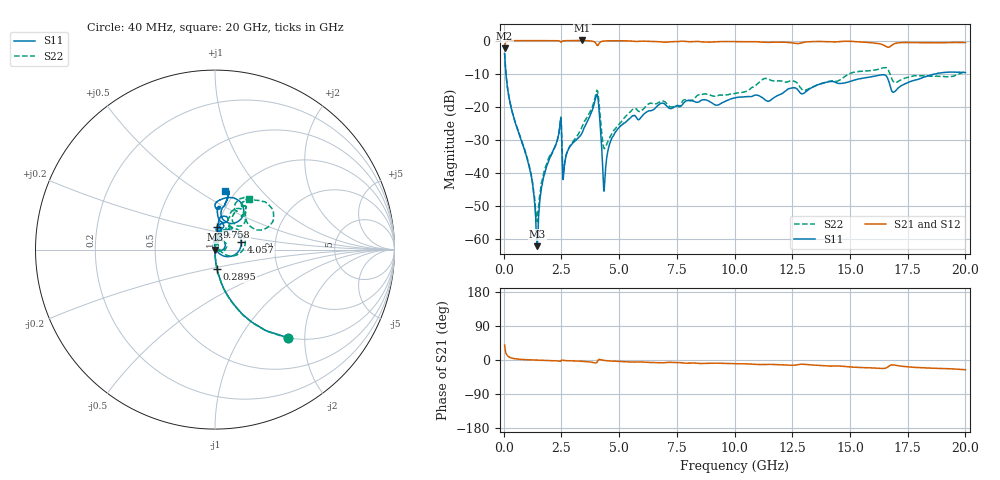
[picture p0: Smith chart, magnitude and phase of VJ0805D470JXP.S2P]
! VJ0805D470JXP
! DATE 10/29/2021  12:48
! CAPACITORS MOUNTED IN SERIES ON 25 MIL THICK MICROSTRIP SUBSTRATE
# GHz  S  MA  R  50.00
!  FREQ  S11M  S11A  S21M  S21A  S12M  S12A  S22M  S22A
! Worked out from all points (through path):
!   1601 points, 40 MHz to 20 GHz, reference 50 ohm
!   highest |S21| = 0.04 dB at 3.408 GHz (marker M1); lowest = -2.3 dB at 40 MHz (marker M2)
!   group delay of S21, straight-line fit = 3.63 ps
!   lowest |S11| = -62.0 dB at 1.462 GHz (marker M3), VSWR 1.00, Z = 49.9 + j0.0319 ohm
!   |S11| at or under -10 dB: 99.02 MHz to 18.74 GHz (18.64 GHz wide, 198 % of centre)
!   |S22| runs from -54.6 to -3.9 dB; largest |S21 - S12| = 0.009
!   S11 on the Smith chart (normalised r, x): 40 MHz: 1.00, -1.66; 289.5 MHz: 1.00, -0.22; 4.057 GHz: 1.34, +0.11; 9.758 GHz: 0.99, +0.26; 20 GHz: 0.89, +0.65
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0.04  0.6375 -50.4  0.7699 39.6  0.767 39.5  0.6402 -50.4
0.2895  0.1085 -84.3  0.9939 6.2  0.9937 6.2  0.1103 -84.0
1.11285  0.01212 -92.9  0.9997 0.4  0.9993 0.4  0.01274 -84.8
1.46215  0.0007928 156.2  0.9989 -0.4  0.9995 -0.4  0.002111 22.7
1.7366  0.008908 92.6  0.9988 -0.9  0.9983 -1.0  0.01002 72.7
2.397775  0.04156 84.8  0.9914 -2.9  0.9921 -3.0  0.04161 71.7
2.6348  0.01356 84.5  0.9962 -1.4  0.997 -1.5  0.01388 65.2
3.370825  0.03887 97.9  1.005 -3.4  1.004 -3.5  0.04781 91.7
3.40825  0.0413 99.4  1.005 -3.5  1.004 -3.7  0.05152 90.9
4.05695  0.1519 15.6  0.8429 -4.1  0.8434 -4.2  0.1763 17.1
4.293975  0.01097 -33.6  0.9798 -0.5  0.9798 -0.7  0.02902 -7.6
4.368825  0.006615 64.1  0.9865 -1.3  0.9868 -1.4  0.02351 23.2
4.593375  0.02812 93.2  0.9936 -2.5  0.9936 -2.6  0.03441 61.6
4.917725  0.04542 90.1  0.9948 -3.6  0.9947 -3.7  0.05065 72.9
6.70165  0.1064 76.4  0.9659 -7.2  0.9664 -7.3  0.1164 59.4
9.758025  0.1288 85.0  0.9673 -9.2  0.9677 -9.4  0.154 58.7
10.02  0.1364 82.5  0.9649 -9.7  0.9646 -9.9  0.1596 59.9
11.34235  0.1261 70.8  0.939 -11.9  0.9391 -12.1  0.269 56.6
13.35083  0.1953 85.5  0.9649 -13.1  0.9655 -13.4  0.1974 61.1
16.68165  0.2431 50.3  0.7932 -16.6  0.7943 -17.0  0.3473 24.9
16.98105  0.1749 75.8  0.9113 -14.0  0.912 -14.4  0.2332 38.5
20  0.3289 80.3  0.9328 -25.7  0.9333 -26.0  0.3401 56.2
